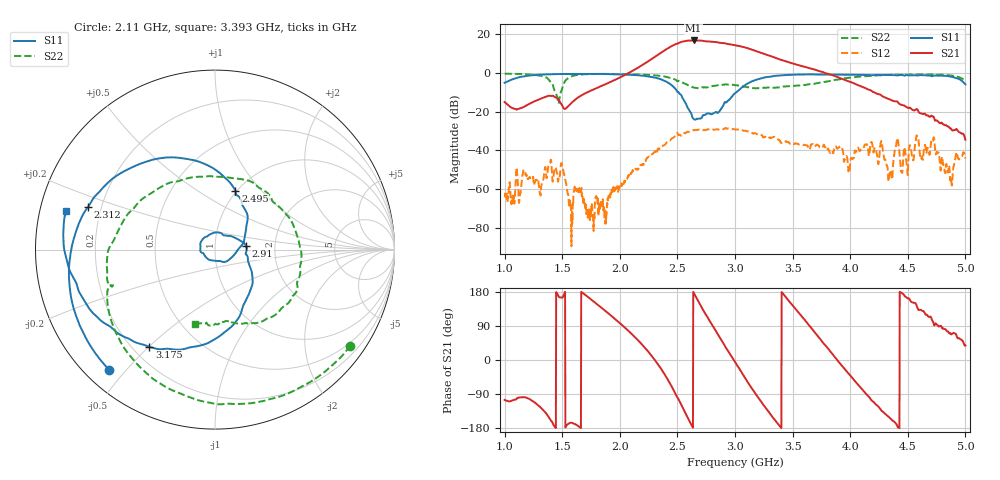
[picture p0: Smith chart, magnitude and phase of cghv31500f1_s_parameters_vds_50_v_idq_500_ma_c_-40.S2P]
!Keysight Technologies,E5071C,MY46632031,B.14.03
!Date: Fri Jul 09 14:58:49 2021
!Data & Calibration Information:
!Freq	S11:SOLT2(ON)	S21:SOLT2(ON)	S12:SOLT2(ON)	S22:SOLT2(ON)
!PortZ  Port1:50+j0  Port2:50+j0
!Above PortZ is port z conversion or system Z0 setting when saving the data.
!When reading, reference impedance value at option line is always used.
# Hz S dB R 50
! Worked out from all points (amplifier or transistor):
!   1601 points, 1 GHz to 5 GHz, reference 50 ohm
!   highest |S21| = 16.8 dB at 2.64 GHz (marker M1)
!   |S21| within 3 dB of that: 2.447 GHz to 3.046 GHz (598.7 MHz wide, 21.8 % of centre)
!   unconditionally stable (mu >= 1): start of sweep to end of sweep
!   at 1.665 GHz: K = 33.87, MAG = 6.2 dB, |S12| = -60.6 dB
!   at 3 GHz: K = 1.84, MAG = 16.4 dB, |S12| = -29.0 dB
!   at 5 GHz: K = 1934.13, MAG = -31.0 dB, |S12| = -44.3 dB
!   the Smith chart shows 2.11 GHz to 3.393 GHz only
!   S11 on the Smith chart (normalised r, x): 2.11 GHz: 0.07, -0.45; 2.312 GHz: 0.15, +0.16; 2.495 GHz: 0.99, +0.73; 2.91 GHz: 1.42, +0.06; 3.175 GHz: 0.27, -0.50; 3.393 GHz: 0.08, +0.13
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1e9  -5.06 152.1  -15.02 -105.3  -62.72 -177.3  -0.36 120.5
1.6675e9  -0.46 -18.3  -11.56 179.4  -59.40 -65.8  -0.78 51.2
2.11e9  -0.99 -131.3  1.08 66.7  -50.74 -12.8  -0.67 -35.4
2.3125e9  -2.54 161.5  8.61 -3.4  -40.63 -94.1  -1.30 -85.3
2.335e9  -2.88 152.8  9.54 -12.7  -39.30 -99.1  -1.39 -92.5
2.42e9  -5.04 113.5  12.86 -53.6  -35.36 -138.2  -2.24 -123.7
2.495e9  -9.21 70.8  15.13 -96.4  -31.39 179.6  -3.97 -160.1
2.5575e9  -14.22 29.1  16.36 -132.9  -31.03 140.7  -5.30 166.4
2.64e9  -23.66 -76.2  16.82 178.3  -29.55 95.0  -7.41 111.3
2.7125e9  -23.00 -164.6  16.70 137.6  -29.38 52.5  -7.38 63.5
2.775e9  -20.95 133.8  16.29 105.9  -29.05 23.4  -7.19 29.3
2.835e9  -20.18 74.9  15.98 75.8  -29.13 -6.3  -6.52 2.7
2.91e9  -15.17 6.9  15.43 38.5  -28.65 -39.4  -5.97 -24.0
3e9  -10.50 -48.6  14.34 -5.3  -29.05 -88.5  -6.27 -51.7
3.09e9  -6.17 -88.5  13.18 -48.5  -29.81 -132.3  -7.15 -70.1
3.175e9  -3.70 -124.1  11.48 -87.9  -31.09 -171.7  -7.88 -80.4
3.2775e9  -2.10 -159.8  9.37 -131.1  -33.58 146.5  -7.53 -91.1
3.3925e9  -1.34 165.6  6.91 -176.3  -35.56 93.5  -7.33 -104.9
3.6675e9  -0.75 96.1  2.17 82.6  -36.82 9.1  -5.66 -151.8
3.99e9  -0.90 19.3  -4.40 -37.0  -49.46 -95.5  -2.47 136.0
4.335e9  -1.01 -73.6  -13.52 -150.3  -55.47 174.4  -1.01 54.3
5e9  -5.87 111.3  -34.51 38.3  -44.27 -24.8  -3.99 -62.4
